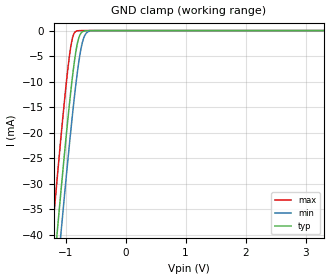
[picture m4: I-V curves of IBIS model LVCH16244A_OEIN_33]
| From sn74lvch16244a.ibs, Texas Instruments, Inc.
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[Model]   LVCH16244A_OEIN_33
Model_type  Input
Vinl=0.8
Vinh=2.0
| variable   typ   min   max
C_comp   3.53pF   2.68pF   4.80pF
[Temperature Range]   40   100   -40
| Ambient temperature   25   85   -40
[Voltage range]   3.3   3   3.6
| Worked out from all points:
|   GND clamp passes 1 mA (typ) near -0.77 V on its own axis
[GND Clamp]
| LVCH16244A_OEIN_33
|   Voltage   I(typ)   I(min)   I(max)
-5V       -583.8mA   -590.8mA   -575.1mA
-1.215V   -49.6mA    -57.88mA   -38.96mA
-1.14V    -39.72mA   -48.01mA   -29.07mA
-1.08V    -31.98mA   -40.25mA   -21.38mA
-1.06V    -29.44mA   -37.69mA   -18.89mA
-925mV    -13.29mA   -21.11mA   -4.122mA
-875mV    -8.124mA   -15.45mA   -1.065mA
-820mV    -3.579mA   -9.774mA   -109.4uA
-770mV    -1.128mA   -5.445mA   -10.73uA
-715mV    -205.4uA   -2.128mA   -808.5nA
-590mV    -2.7uA     -81.86uA   -2.255nA
3.3V      6.304pA    9.258pA    5.93pA
